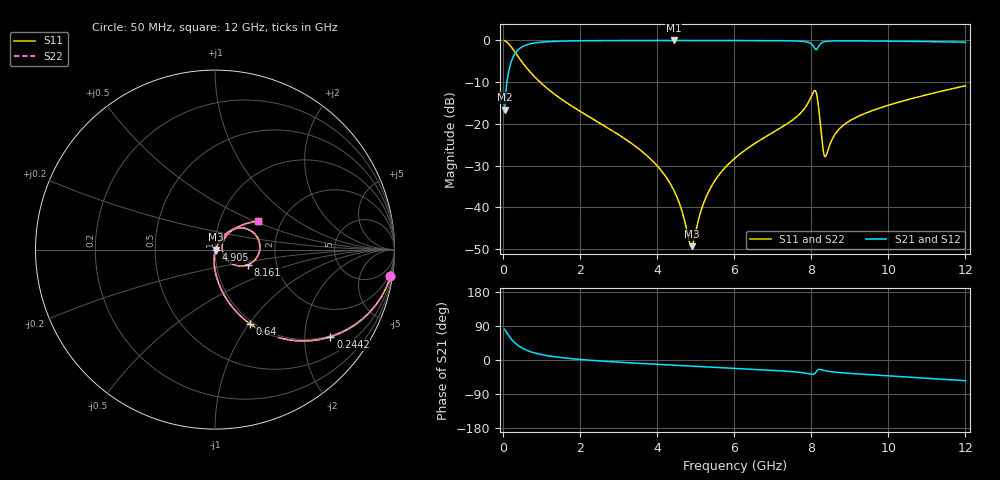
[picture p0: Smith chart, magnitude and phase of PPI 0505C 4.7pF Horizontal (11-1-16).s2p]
# MHz S MA R 50
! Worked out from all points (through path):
!   1601 points, 50 MHz to 12 GHz, reference 50 ohm
!   highest |S21| = -0.03 dB at 4.442 GHz (marker M1); lowest = -16.6 dB at 50 MHz (marker M2)
!   group delay of S21, straight-line fit = 18 ps
!   lowest |S11| = -49.3 dB at 4.897 GHz (marker M3), VSWR 1.01, Z = 50.3 - j0.0911 ohm
!   |S11| at or under -10 dB: 967.7 MHz to end of sweep
!   |S22| runs from -49.3 to -0.1 dB; largest |S21 - S12| = 0
!   S11 on the Smith chart (normalised r, x): 50 MHz: 1, -13; 244.2 MHz: 0.96, -2.68; 640 MHz: 0.97, -1.01; 4.905 GHz: 1.01, -0.00; 8.161 GHz: 1.43, -0.25; 12 GHz: 1.52, +0.52
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50  0.9889 -8.7  0.1482 81.3  0.1482 81.3  0.9889 -8.7
154.5625  0.9071 -25.4  0.4206 64.6  0.4206 64.6  0.9071 -25.4
244.1875  0.8061 -37.1  0.5912 52.9  0.5912 52.9  0.8061 -37.1
430.9062  0.6094 -53.8  0.792 36.1  0.792 36.1  0.6094 -53.8
640.0312  0.4567 -64.8  0.8884 25.1  0.8884 25.1  0.4567 -64.8
1125.5  0.2725 -77.6  0.9605 12.1  0.9605 12.1  0.2725 -77.6
2044.156  0.1379 -88.0  0.9882 1.2  0.9882 1.2  0.1379 -88.0
4038.312  0.03023 -95.8  0.9963 -11.5  0.9963 -11.5  0.03023 -95.8
4441.625  0.0159 -92.1  0.9964 -13.7  0.9964 -13.7  0.0159 -92.1
4897.219  0.003422 -15.3  0.9963 -16.0  0.9963 -16.0  0.003422 -15.3
4904.688  0.003438 -11.2  0.9963 -16.1  0.9963 -16.1  0.003438 -11.2
5345.344  0.01557 58.0  0.9959 -18.3  0.9959 -18.3  0.01557 58.0
6025  0.03882 62.0  0.9947 -21.9  0.9947 -21.9  0.03882 62.0
7593.438  0.1183 53.8  0.9826 -31.4  0.9826 -31.4  0.1183 53.8
8019.156  0.2207 29.8  0.8941 -37.7  0.8941 -37.7  0.2207 29.8
8101.312  0.2508 3.4  0.7911 -35.2  0.7911 -35.2  0.2508 3.4
8161.062  0.2027 -24.4  0.7969 -26.9  0.7969 -26.9  0.2027 -24.4
8302.969  0.05166 -26.6  0.9478 -26.8  0.9478 -26.8  0.05166 -26.6
8370.188  0.04059 9.5  0.9672 -28.5  0.9672 -28.5  0.04059 9.5
8855.656  0.09777 50.7  0.9858 -34.1  0.9858 -34.1  0.09777 50.7
10013.31  0.1675 45.9  0.9784 -41.7  0.9784 -41.7  0.1675 45.9
12000  0.2854 33.6  0.9493 -54.7  0.9493 -54.7  0.2854 33.6
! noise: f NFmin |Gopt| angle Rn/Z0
50  0.0005192  0.9082  2.175  0.001242
1372  0.004906  0.7273  5.194  0.00357
2701  0.008124  0.6843  9.274  0.004958
4031  0.01111  0.6616  13.38  0.006198
5360  0.01417  0.6514  17.44  0.00756
6682  0.01808  0.6601  21.42  0.00983
8012  0.08155  0.8977  25.85  0.1654
9341  0.02573  0.6707  29.44  0.0141
1.067e+04  0.02786  0.6592  33.04  0.01441
1.2e+04  0.03203  0.6692  36.66  0.01684
